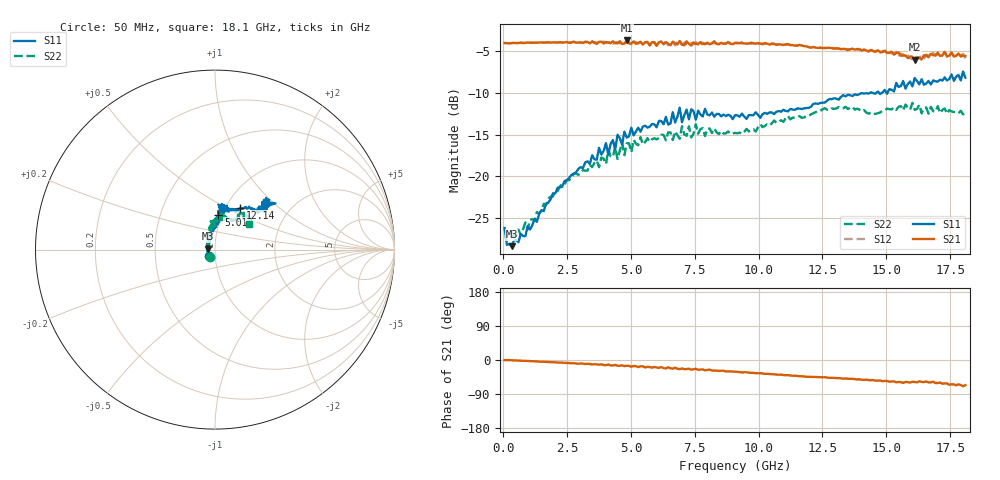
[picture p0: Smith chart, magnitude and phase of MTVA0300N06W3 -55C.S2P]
! Network Analyzer HP8720D.06.14 Serial No. US36140669
!  7 Jul 2005  10:09:29
! Frequency  S11  S21  S12  S22
# HZ  S  DB R 50
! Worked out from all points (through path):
!   201 points, 50 MHz to 18.1 GHz, reference 50 ohm
!   highest |S21| = -3.74 dB at 4.833 GHz (marker M1); lowest = -6.0 dB at 16.11 GHz (marker M2)
!   group delay of S21, straight-line fit = 10.4 ps
!   lowest |S11| = -28.3 dB at 320.8 MHz (marker M3), VSWR 1.08, Z = 46.3 + j0.434 ohm
!   |S11| at or under -10 dB: start of sweep to 14.37 GHz; 14.45 GHz to 14.61 GHz (167.7 MHz wide, 1.15 % of centre); 14.72 GHz to 14.83 GHz (113 MHz wide, 0.765 % of centre)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
!   |S22| runs from -27.2 to -11.2 dB; largest |S21 - S12| = 0.036
!   S11 on the Smith chart (normalised r, x): 50 MHz: 0.93, -0.06; 5.014 GHz: 0.96, +0.39; 12.14 GHz: 1.17, +0.59; 18.1 GHz: 1.47, +0.91
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5e7  -26.16 -135.7  -4.05 -0.2  -4.06 -0.3  -26.29 -122.7
1.4025e8  -28.18 -165.4  -4.06 -0.4  -4.05 -0.4  -27.12 -164.2
3.2075e8  -28.34 173.0  -4.06 -0.8  -4.06 -0.8  -26.76 175.1
9.525e8  -25.93 135.5  -3.98 -2.6  -4.02 -2.5  -26.33 144.0
3.1185e9  -19.00 94.6  -4.04 -9.5  -4.05 -10.0  -19.22 106.6
4.47225e9  -15.02 81.3  -4.08 -15.1  -3.94 -13.5  -17.91 100.5
4.65275e9  -16.20 81.2  -4.16 -14.2  -3.90 -15.5  -15.94 98.6
4.743e9  -14.64 83.8  -4.11 -16.0  -4.08 -14.6  -17.46 94.7
4.83325e9  -15.36 89.3  -3.74 -15.3  -3.99 -16.7  -16.04 87.8
5.01375e9  -14.16 84.6  -4.14 -17.8  -4.23 -16.2  -17.09 90.0
5.104e9  -15.09 86.1  -3.85 -15.9  -3.93 -17.3  -15.62 89.7
6.09675e9  -13.35 80.4  -3.95 -20.7  -3.89 -20.3  -15.42 85.2
6.7285e9  -13.56 85.1  -4.07 -20.3  -4.33 -21.7  -14.61 78.0
6.909e9  -11.77 81.5  -3.81 -24.3  -4.00 -22.3  -15.49 77.3
6.99925e9  -13.52 81.3  -4.18 -22.2  -4.28 -24.7  -13.99 77.6
7.17975e9  -12.01 85.7  -3.84 -23.9  -4.19 -22.9  -15.13 72.5
7.54075e9  -13.21 76.7  -4.15 -23.2  -3.95 -26.1  -13.77 80.0
9.075e9  -12.68 77.6  -4.05 -30.8  -4.02 -30.9  -14.78 66.3
1.21435e10  -11.32 58.5  -4.54 -44.5  -4.50 -44.5  -12.44 55.7
1.512175e10  -9.57 40.2  -5.22 -57.4  -4.99 -56.7  -11.96 46.9
1.61145e10  -8.24 39.1  -6.05 -58.2  -5.59 -58.0  -12.03 43.2
1.81e10  -8.20 42.5  -5.59 -66.5  -5.88 -67.3  -12.52 36.9
